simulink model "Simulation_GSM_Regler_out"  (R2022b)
settings: Solver=ode15s  StartTime=0.0  StopTime=15  MaxStep=1e-2  RelTol=1e-7  AbsTol=1e-5  EnableMultiTasking=on
undefined symbols (not defined in the file or in its folder): A, B, C, D, parGSM, x0
libraries: cstblocks x3

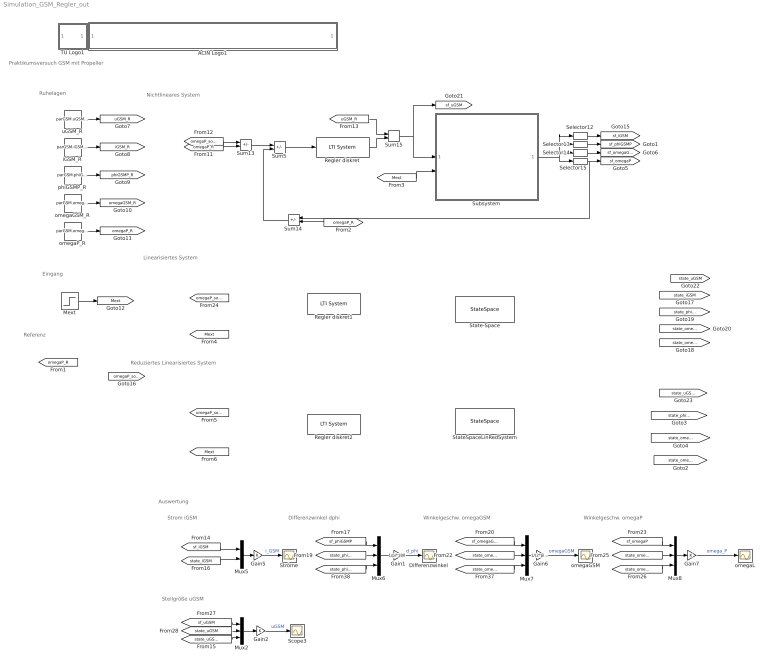
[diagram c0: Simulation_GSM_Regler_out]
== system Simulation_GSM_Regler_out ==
  note: Referenz
  note: Eingang
  note: Ruhelagen
  note: Auswertung
  note: Nichtlineares System
  note: Linearisiertes System
  note: Reduziertes Linearisiertes System
  note: Differenzwinkel dphi
  note: Winkelgeschw. omegaGSM
  note: Winkelgeschw. omegaP
  note: Praktikumsversuch GSM mit Propeller
  note: Strom iGSM
  note: Stellgröße uGSM
  ACIN Logo1 : Subsystem
      mask init:
      | s = get_param(gcb,'UserData');
  Differenzwinkel : Scope
  Gain1 : Gain  Gain=1/pi*180
  Gain2 : Gain
  Gain5 : Gain
  Gain6 : Gain  Gain=1/(2*pi)*60
  Gain7 : Gain
  Mext : Step  Time=11  After=0.25  SampleTime=0
  Mux{2,6..8} (4 alike) : Mux  Inputs=3
  Mux5 : Mux  Inputs=2
  Regler diskret : cstblocks/LTI System  sys=KompReg  IC=[]
  Regler diskret1 : cstblocks/LTI System  sys=KompReg  IC=[]
  Regler diskret2 : cstblocks/LTI System  sys=KompReg  IC=[]
  Scope3 : Scope
  Selector12 : Selector  InputPortWidth=4  IndexOptions=Index vector (dialog)  Indices=[1]  OutputSizes=1
  Selector13 : Selector  InputPortWidth=4  IndexOptions=Index vector (dialog)  Indices=[2]  OutputSizes=1
  Selector14 : Selector  InputPortWidth=4  IndexOptions=Index vector (dialog)  Indices=[3]  OutputSizes=1
  Selector15 : Selector  InputPortWidth=4  IndexOptions=Index vector (dialog)  Indices=[4]  OutputSizes=1
  State-Space : StateSpace  A=A  B=B  C=C  D=D  InitialCondition=x0
  StateSpaceLinRedSystem : StateSpace  A=A  B=B  C=C  D=D  InitialCondition=x0
  Ströme : Scope
  Subsystem : Subsystem
  Sum13 : Sum  Inputs=+-
  Sum14 : Sum  Inputs=+-
  Sum15 : Sum
  Sum5 : Sum  Inputs=+-
  TU Logo1 : Subsystem
      mask init:
      | s = get_param(gcb,'UserData');
  iGSM_R : Constant  Value=parGSM.iGSM_R
  omegaGSM : Scope
  omegaGSM_R : Constant  Value=parGSM.omegaGSM_R
  omegaL : Scope
  omegaP_R : Constant  Value=parGSM.omegaP_R
  phiGSMP_R : Constant  Value=parGSM.phiGSMP_R
  uGSM_R : Constant  Value=parGSM.uGSM_R
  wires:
  Mux5/1 -> Gain5/1
  Gain5/1 -> Ströme/1  "i_GSM"
  [sf_iGSM] -> Mux5/1
  Mux6/1 -> Gain1/1
  Gain1/1 -> Differenzwinkel/1  "d_phi"
  [sf_phiGSMP] -> Mux6/1
  Mux7/1 -> Gain6/1
  Gain6/1 -> omegaGSM/1  "omegaGSM"
  Mux8/1 -> Gain7/1
  Gain7/1 -> omegaL/1  "omega_P"
  [sf_omegaP] -> Mux8/1
  [state_phiGSMP] -> Mux6/2
  [state_phiGSMPred] -> Mux6/3
  [state_omegaP] -> Mux8/2
  [state_omegaPred] -> Mux8/3
  [state_iGSM] -> Mux5/2
  [sf_omegaGSM] -> Mux7/1
  [state_omegaGSM] -> Mux7/2
  [state_omegaGSMred] -> Mux7/3
  [Mext] -> Subsystem/2(Mext)
  Subsystem/1(y) -> Selector12/1, Selector13/1, Selector14/1, Selector15/1
  Selector13/1 -> [sf_phiGSMP]
  Selector12/1 -> [sf_iGSM]
  Selector14/1 -> [sf_omegaGSM]
  omegaGSM_R/1 -> [omegaGSM_R]
  omegaP_R/1 -> [omegaP_R]
  phiGSMP_R/1 -> [phiGSMP_R]
  iGSM_R/1 -> [iGSM_R]
  uGSM_R/1 -> [uGSM_R]
  Mext/1 -> [Mext]
  [omegaP_R] -> Sum13/2
  [omegaP_soll] -> Sum13/1
  Sum13/1 -> Sum5/1
  Sum5/1 -> Regler diskret/1
  Sum14/1 -> Sum5/2
  [omegaP_R] -> Sum14/2
  Selector15/1 -> Sum14/1, [sf_omegaP]
  Sum15/1 -> Subsystem/1(uGSM), [sf_uGSM]
  Regler diskret/1 -> Sum15/2
  [uGSM_R] -> Sum15/1
  Mux2/1 -> Gain2/1
  Gain2/1 -> Scope3/1  "uGSM"
  [state_uGSMred] -> Mux2/3
  [state_uGSM] -> Mux2/2
  [sf_uGSM] -> Mux2/1

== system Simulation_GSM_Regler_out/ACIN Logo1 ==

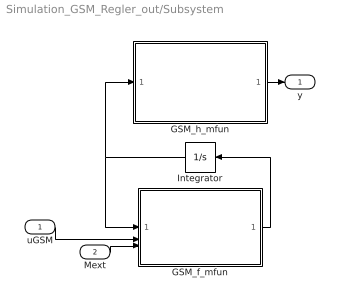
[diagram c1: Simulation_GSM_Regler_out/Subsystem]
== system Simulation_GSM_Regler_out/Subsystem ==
  uGSM : Inport
  Mext : Inport  Port=2
  GSM_f_mfun : MATLAB Function  TreatAsAtomicUnit=on
  GSM_h_mfun : MATLAB Function  TreatAsAtomicUnit=on
  Integrator : Integrator  InitialCondition=[parGSM.iGSM_R;parGSM.phiGSMP_R;parGSM.omegaGSM_R;parGSM.omegaP_R]
  y : Outport
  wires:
  GSM_f_mfun/1(dx) -> Integrator/1
  uGSM/1 -> GSM_f_mfun/2(u1)
  GSM_h_mfun/1(y) -> y/1
  Integrator/1 -> GSM_f_mfun/1(x), GSM_h_mfun/1(x)
  Mext/1 -> GSM_f_mfun/3(u2)

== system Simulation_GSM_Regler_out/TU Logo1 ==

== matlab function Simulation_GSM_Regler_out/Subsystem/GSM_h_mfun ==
function y = GSM_h_mfun(x,parGSM)
%To DO
return;

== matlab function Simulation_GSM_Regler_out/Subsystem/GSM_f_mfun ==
function dx = GSM_f_mfun(x,u1,u2,parGSM)
%To Do
return;
